(* Logix 5000 DataType export UDT_ISC_OutDataConversion; software revision 32.02 *)

TYPE UDT_ISC_OutDataConversion :
STRUCT
   ProductDest : INT;   // Destination for next product to be inducted - ISC CAM set for internal mode
   RunModeInternal : BOOL;   // Run mode internal - ISC CAM balancing logic control
   RunModeExternal : BOOL;   // Run mode external - PLC balancing logic control
   QuantityLane0 : INT;   // Quantity of products to destination 0 for line balancing - ISC CAM internal mode
   QuantityLane1 : INT;   // Quantity of products to destination 1 for line balancing - ISC CAM internal mode
   QuantityLane2 : INT;   // Quantity of products to destination 2 for line balancing - ISC CAM internal mode
   QuantityLane3 : INT;   // Quantity of products to destination 3 for line balancing - ISC CAM internal mode
   QuantityLane4 : INT;   // Quantity of products to destination 4 for line balancing - ISC CAM internal mode
   QuantityLane5 : INT;   // Quantity of products to destination 5 for line balancing - ISC CAM internal mode
   QuantityLane6 : INT;   // Quantity of products to destination 6 for line balancing - ISC CAM internal mode
   EnableLeftCarryway1 : BOOL;   // Enable/Disable carryway 1 left 0 = Disable 1 = Enable
   EnableRightCarryway1 : BOOL;   // Enable/Disable carryway 1 right 0 = Disable 1 = Enable
   EnableLeftCarryway2 : BOOL;   // Enable/Disable carryway 2 left 0 = Disable 1 = Enable
   EnableRightCarryway2 : BOOL;   // Enable/Disable carryway 2 right 0 = Disable 1 = Enable
   EnableLeftCarryway3 : BOOL;   // Enable/Disable carryway 3 left 0 = Disable 1 = Enable
   EnableRightCarryway3 : BOOL;   // Enable/Disable carryway 3 right 0 = Disable 1 = Enable
   OverrideCarrywayPointer : INT;   // Override active carryway point value
   ParameterGroupWrite : INT;   // Parameter group number write - 1, 2, 3, 6, or 7
   ParameterRead : BOOL;   // Parameter read value trigger
   ParameterWrite : BOOL;   // Parameter write value trigger
END_STRUCT
END_TYPE
